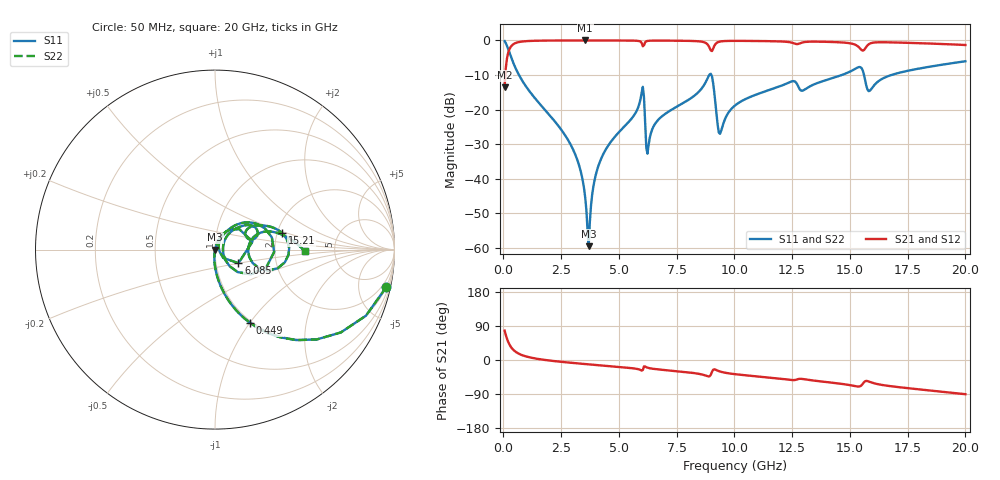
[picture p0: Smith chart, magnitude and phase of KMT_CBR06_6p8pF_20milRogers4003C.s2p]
! Data measured by Modelithics Inc. support@modelithics.com 813-866-6335
! KEMET CBR0603 6.8pF, Pad Width= 0.851mm, Pad Length= 0.64mm, Pad Gap= 0.62mm, 20mil Rogers 4003C substrate Data, January 2022
# hz S ma R 50
! 2 Port Network Data from SP1.SP block
! freq  magS11  angS11  magS21  angS21  magS12  angS12  magS22  angS22
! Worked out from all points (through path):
!   401 points, 50 MHz to 20 GHz, reference 50 ohm
!   highest |S21| = -0.01 dB at 3.541 GHz (marker M1); lowest = -13.5 dB at 50 MHz (marker M2)
!   group delay of S21, straight-line fit = 13.9 ps
!   lowest |S11| = -59.4 dB at 3.691 GHz (marker M3), VSWR 1.00, Z = 50.1 + j0.0136 ohm
!   |S11| at or under -10 dB: 673.6 MHz to 8.91 GHz (8.236 GHz wide, 172 % of centre); 9.002 GHz to 14.64 GHz (5.641 GHz wide, 47.7 % of centre); 15.61 GHz to 16.79 GHz (1.179 GHz wide, 7.28 % of centre)
!   |S22| runs from -59.4 to -0.2 dB; largest |S21 - S12| = 0
!   S11 on the Smith chart (normalised r, x): 50 MHz: 0.98, -9.16; 449 MHz: 0.98, -1.01; 6.085 GHz: 1.28, -0.20; 15.21 GHz: 2.13, +0.45; 20 GHz: 3.00, -0.07
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5e7  0.9775 -12.3  0.2108 77.7  0.2108 77.7  0.9775 -12.3
2.495e8  0.6789 -48.0  0.7338 42.0  0.7338 42.0  0.6789 -48.0
4.49e8  0.4535 -64.4  0.8907 25.6  0.8907 25.6  0.4535 -64.4
2.793125e9  0.03664 -95.2  0.9984 -6.6  0.9984 -6.6  0.03664 -95.2
3.391625e9  0.01104 -94.9  0.9989 -9.9  0.9989 -9.9  0.01104 -94.9
3.54125e9  0.005333 -90.0  0.9989 -10.7  0.9989 -10.7  0.005333 -90.0
3.690875e9  0.001067 7.3  0.9989 -11.5  0.9989 -11.5  0.001067 7.3
3.94025e9  0.009421 70.8  0.9988 -12.8  0.9988 -12.8  0.009421 70.8
4.289375e9  0.02166 72.5  0.9985 -14.5  0.9985 -14.5  0.02166 72.5
5.985125e9  0.1768 40.2  0.9204 -28.0  0.9204 -28.0  0.1768 40.2
6.084875e9  0.151 -29.9  0.8521 -16.9  0.8521 -16.9  0.151 -29.9
6.284375e9  0.03097 47.7  0.9882 -21.1  0.9882 -21.1  0.03097 47.7
6.73325e9  0.0732 62.6  0.9941 -25.0  0.9941 -25.0  0.0732 62.6
8.92775e9  0.324 12.2  0.7783 -42.9  0.7783 -42.9  0.324 12.2
9.376625e9  0.04476 7.3  0.9639 -30.4  0.9639 -30.4  0.04476 7.3
1.0025e10  0.1148 48.8  0.9854 -37.4  0.9854 -37.4  0.1148 48.8
1.336662e10  0.2254 32.7  0.9601 -53.8  0.9601 -53.8  0.2254 32.7
1.5212e10  0.3858 13.6  0.8719 -68.7  0.8719 -68.7  0.3858 13.6
1.5611e10  0.3176 -21.5  0.7273 -58.4  0.7273 -58.4  0.3176 -21.5
1.586038e10  0.1873 4.6  0.8985 -57.7  0.8985 -57.7  0.1873 4.6
1.670825e10  0.3095 19.1  0.9381 -68.7  0.9381 -68.7  0.3095 19.1
2e10  0.5002 -1.0  0.8584 -90.2  0.8584 -90.2  0.5002 -1.0
